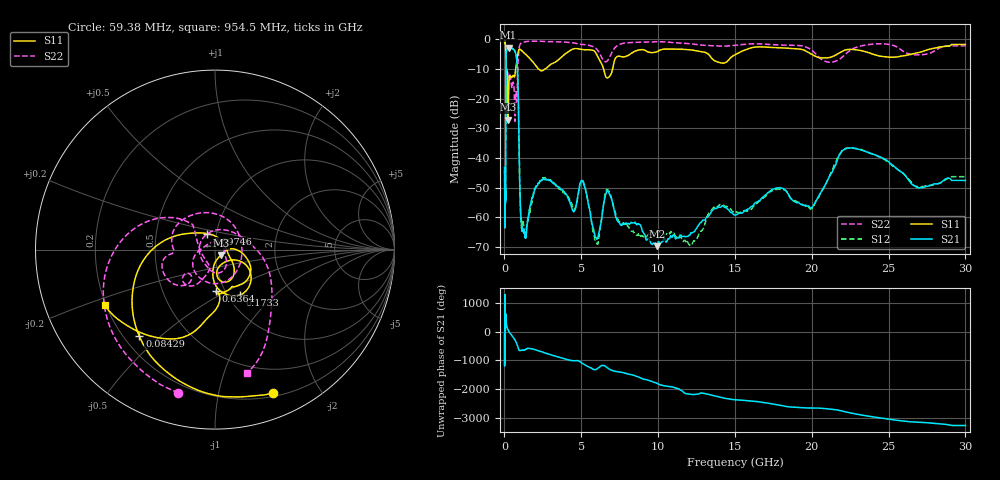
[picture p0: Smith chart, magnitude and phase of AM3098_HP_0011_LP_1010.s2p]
! Date/Time: Thu, Feb 28, 2019 8:34 AM
! Network Analyzer: Agilent Technologies E8364B Rev: A.07.50.67
! Sweep from 0.010 to 30.000 GHz, 1601 Points, Sweep Type: LOG
! Power Supply: 5.022 V, 0.002 A
# Hz S DB R 50
!freq MagS11 AngS11 MagS21 AngS21 MagS12 AngS12 MagS22 AngS22
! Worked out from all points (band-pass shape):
!   1601 points, 10 MHz to 30 GHz, reference 50 ohm
!   highest |S21| = -2.80 dB at 266.5 MHz (marker M1); lowest = -69.8 dB at 9.928 GHz (marker M2)
!   |S21| within 3 dB of the highest: 108.7 MHz to 772.4 MHz (663.7 MHz wide, 151 % of centre)
!   lowest |S11| = -27.1 dB at 233.9 MHz (marker M3), VSWR 1.09, Z = 53.1 - j3.3 ohm
!   |S11| at or under -10 dB: 93.01 MHz to 730.6 MHz (637.6 MHz wide, 155 % of centre); 2.225 GHz to 2.651 GHz (426.3 MHz wide, 17.5 % of centre); 6.454 GHz to 7.039 GHz (584.6 MHz wide, 8.67 % of centre)
!   |S22| runs from -27.7 to -0.6 dB; largest |S21 - S12| = 0.013
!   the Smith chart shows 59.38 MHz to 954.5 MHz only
!   S11 on the Smith chart (normalised r, x): 59.38 MHz: 0.23, -1.46; 84.29 MHz: 0.26, -0.43; 97.46 MHz: 0.90, +0.16; 173.3 MHz: 1.14, -0.63; 636.4 MHz: 0.91, -0.45; 954.5 MHz: 0.20, -0.23
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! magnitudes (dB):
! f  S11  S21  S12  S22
! 10 MHz  -0.3  -43.2  -43.8  -0.6
! 38.04 MHz  -0.5  -61.1  -60.3  -1.0
! 59.38 MHz  -1.3  -53.5  -51.9  -1.7
! 73.27 MHz  -2.0  -53.4  -54.6  -2.5
! 84.29 MHz  -3.9  -34.4  -34.2  -4.3
! 97.46 MHz  -20.0  -10.8  -10.7  -21.8
! 144.7 MHz  -15.5  -3.5  -3.5  -13.1
! 173.3 MHz  -10.8  -3.4  -3.3  -10.1
! 233.9 MHz  -27.1  -2.9  -2.9  -12.5
! 266.5 MHz  -17.6  -2.8  -2.8  -12.8
! 550.5 MHz  -12.2  -3.3  -3.2  -14.5
! 636.4 MHz  -12.7  -3.6  -3.6  -17.9
! 838.1 MHz  -5.8  -9.5  -9.4  -14.9
! 954.5 MHz  -3.3  -37.4  -37.3  -3.0
! 1.076 GHz  -3.6  -60.2  -60.5  -1.3
! 1.328 GHz  -4.8  -66.5  -66.3  -0.8
! 2.084 GHz  -9.2  -49.4  -49.5  -0.6
! 7.926 GHz  -5.7  -62.0  -61.9  -1.1
! 9.928 GHz  -4.2  -69.8  -65.4  -0.8
! 19.7 GHz  -4.2  -56.4  -56.8  -2.7
! 22.67 GHz  -3.4  -36.7  -36.7  -3.2
! 30 GHz  -1.7  -47.6  -46.3  -2.2
